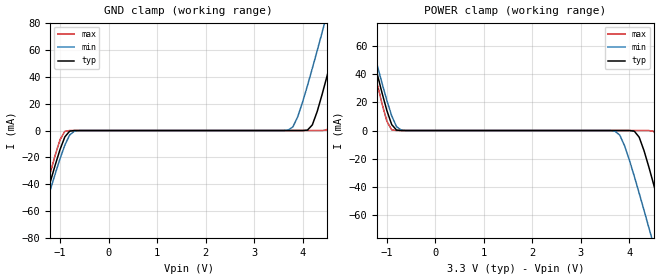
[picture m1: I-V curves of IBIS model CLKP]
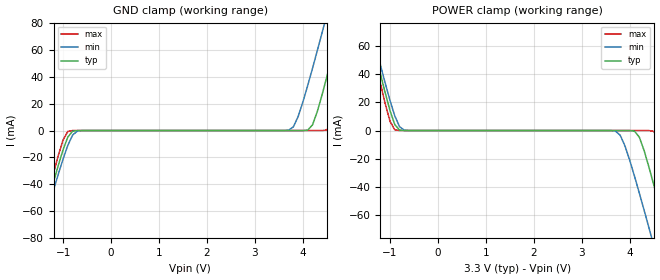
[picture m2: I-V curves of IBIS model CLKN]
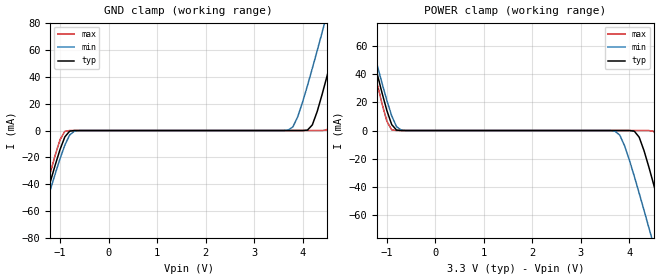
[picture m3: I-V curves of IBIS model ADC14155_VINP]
|   National Semiconductor Corporation
|   IBIS Model of ADC14155_qml
|   48 Pin LLP
[IBIS Ver]   4.0
[File name]   adc14155_qml.ibs
[File Rev]   1.0
[Date]   07/15/2009
[Source]
[Notes]   Revision History:
   Revision 1.0 : Models Generated by Shrikant GK
   Revision 1.1 : Added QML package to the IBIS file Pegah Alavi
[Disclaimer]
(C) Copyright National Semiconductor Corporation 2009
   All rights reserved
   National Semiconductor Corporation hereby grants
the user of this IBIS model a non-exclusive, nontransferable
license to use this IBIS model under the following terms.
Before using this IBIS model, the user should read this
license.  If the user does not accept these terms,  the
IBIS model should be returned to National within 30 days.
   The user is granted this license only to use the
IBIS model and is not granted rights to sell, load, rent,
lease or license the IBIS model in whole or in part, or in
modified form to anyone other than user. User may modify
the IBIS model to suit its specific applications but rights
to derivative works and such modifications shall belong to
National.
   This IBIS model is provided on an "AS IS" basis and
National makes absolutely no warranty with respect to the
information contained herein.NATIONAL DISCLAIMS AND CUSTOMER
WAIVES ALL WARRANTIES, EXPRESS OR IMPLIED, INCLUDING
WARRANTIES OF MERCHANTABILITY OR FITNESS FOR A PARTICULAR
PURPOSE. The entire risk as to quality and performance is
with the Customer. ACCORDINGLY, IN NO EVENT SHALL THE
COMPANY BE LIABLE FOR ANY DAMAGES, WHETHER IN CONTRACT OR
TORT,INCLUDING ANY LOST PROFITS OR OTHER INCIDENTAL,
CONSEQUENTIAL, EXEMPLARY, OR PUNITIVE DAMAGES ARISING OUT
OF THE USE OR APPLICATION OF THE IBIS model provided in
this package.Further, National reserves the right to make
changes without notice to any product herein to improve
reliability, function, or design. National does not convey
any license under patent rights or any other intellectual
property rights, including those of third parties.
   National is not obligated to provide maintenance or support
for the licensed IBIS model.
[Copyright]   Copyright 2009, National Semiconductor, All Rights Reserved
[Component]   ADC14155_qml
[Manufacturer]  National Semiconductor Corp
[Package]
|   typ   min   max
R_pkg   0   0   0
L_pkg   0   0   0
C_pkg   0   0   0
[Pin]   signal_name  model_name   R_pin   L_pin   C_pin
1   VA   POWER
2   AGND   GND
3   VIN-   ADC14155_VINN
4   VIN+   ADC14155_VINP
5   AGND   GND
6   VA   POWER
7   PD   NC
8   CLK_SEL   NC
9   VA   POWER
10   AGND   GND
11   CLK+   CLKP
12   CLK-   CLKN
13   VD   POWER
14   DGND   GND
15   VDR   POWER
16   DRGND   GND
17   D0   ADC14155_D0
18   D1   ADC14155_D0
19   D2   ADC14155_D0
20   D3   ADC14155_D0
21   D4   ADC14155_D0
22   D5   ADC14155_D0
23   D6   ADC14155_D0
24   D7   ADC14155_D0
25   VDR   POWER
26   DRGND   GND
27   D8   ADC14155_D0
28   D9   ADC14155_D0
29   D10   ADC14155_D0
30   D11   ADC14155_D0
31   D12   ADC14155_D0
32   D13   ADC14155_D0
33   OVR   NC
34   DRDY   ADC14155_D0
35   DRGND   GND
36   VDR   POWER
37   VA   POWER
38   AGND   GND
39   AGND   GND
40   VA   POWER
41   VA   POWER
42   AGND   GND
43   VRP   NC
44   VRN   NC
45   VRM   NC
46   VREF   NC
47   AGND   GND
48   VA   POWER
49   DAP   GND
[Diff_pin]   inv_pin   vdiff   tdelay_typ   tdelay_min   tdelay_max
| The '+' pin is Diff_pin and the '-' pin is the inv_pin
4   3   50m   0   0   0
|Electrical package information will overide all the default values.
[Package Model] ADC14155W_QML
|   Package Model
[Define Package Model]  ADC14155W_QML
[Manufacturer]   NSC
[Description]   none
[OEM]   NA
[Number Of Pins]   21
[Pin Numbers]
10   | 10 = B10
11   | 11 = B11
12   | 12 = B12
17   | 17 = B17
18   | 18 = B18
19   | 19 = B19
20   | 20 = B20
21   | 21 = B21
22   | 22 = B22
23   | 23 = B23
24   | 24 = B24
25   | 25 = B25
26   | 26 = B26
27   | 27 = B27
28   | 28 = B28
30   | 30 = B30
31   | 31 = B31
32   | 32 = B32
33   | 33 = B33
34   | 34 = B34
35   | 35 = B35
[Model Data]
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[End Model Data]
[End Package Model]
| Models and submodels in the file (5): CLKP (Input), CLKN (Input), ADC14155_VINP (Input), ADC14155_VINN (Input), ADC14155_D0 (Output)
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|   Input driver CLKP
[Model]   CLKP
Model_type Input
Polarity Non-Inverting
Vinh=2.0
Vinl=0.8
C_comp   776.6f   764.4f   787.6f
|   TYP   MIN   MAX
[Temperature Range]  25   85   -40
[Voltage Range]   3.3   3.0   3.6
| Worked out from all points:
|   GND clamp passes 1 mA (typ) near -0.81 V on its own axis
|   POWER clamp passes 1 mA (typ) near -0.82 V on its own axis
[GND Clamp]
|V(groundclamp)   I(typ)   I(min)   I(max)
-3.3V     -322.4mA   -312.6mA   -335.1mA
-1.5V     -77.49mA   -81.34mA   -73.54mA
-1.1V     -25.94mA   -32.53mA   -18.6mA
-900mV    -4.742mA   -10.9mA    -604uA
-600mV    -278.4nA   -17.67uA   -369.6pA
3.7V      84.77pA    241.1uA    8.991pA
3.9V      166.1nA    10.36mA    9.951pA
4.2V      4.188mA    46.42mA    221.4pA
4.5V      40.21mA    86.59mA    437.8uA
4.8V      82.74mA    127.8mA    33.34mA
5.1V      126.5mA    169.5mA    78.82mA
6.5V      334.4mA    366.6mA    299.9mA
[POWER Clamp]
|V(PowerClamp)   I(typ)   I(min)   I(max)
-3.3V     349.4mA    338.3mA    315.9mA
-1.5V     82.74mA    86.59mA    78.82mA
-1.4V     68.37mA    73.03mA    63.43mA
-900mV    4.188mA    10.36mA    437.8uA
-700mV    7.783uA    241.1uA    28.92nA
3.7V      -141.7pA   -368.4uA   -7.681pA
3.9V      -278.4nA   -10.9mA    -8.642pA
4.2V      -4.742mA   -44.39mA   -369.6pA
4.5V      -38.39mA   -81.34mA   -604uA
4.8V      -77.49mA   -119.2mA   -31.74mA
5.1V      -117.7mA   -157.5mA   -73.54mA
6.5V      -308.6mA   -312.6mA   -276.5mA
|   Input driver CLKN
[Model]   CLKN
Model_type Input
Polarity Inverting
Vinh=2.0
Vinl=0.8
C_comp   776.6f   764.4f   787.6f
|   TYP   MIN   MAX
[Temperature Range]   25   85   -40
[Voltage Range]   3.3   3.0   3.6
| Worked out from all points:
|   GND clamp passes 1 mA (typ) near -0.81 V on its own axis
|   POWER clamp passes 1 mA (typ) near -0.82 V on its own axis
[GND Clamp]
|V(groundclamp)   I(typ)   I(min)   I(max)
-3.3V     -322.4mA   -312.6mA   -335.1mA
-1.5V     -77.49mA   -81.34mA   -73.54mA
-1.1V     -25.94mA   -32.53mA   -18.6mA
-900mV    -4.742mA   -10.9mA    -604uA
-600mV    -278.4nA   -17.67uA   -369.6pA
3.7V      84.77pA    241.1uA    8.991pA
3.9V      166.1nA    10.36mA    9.951pA
4.2V      4.188mA    46.42mA    221.4pA
4.5V      40.21mA    86.59mA    437.8uA
4.8V      82.74mA    127.8mA    33.34mA
5.1V      126.5mA    169.5mA    78.82mA
6.5V      334.4mA    366.6mA    299.9mA
[POWER Clamp]
|V(PowerClamp)   I(typ)   I(min)   I(max)
-3.3V     349.4mA    338.3mA    315.9mA
-1.5V     82.74mA    86.59mA    78.82mA
-1.4V     68.37mA    73.03mA    63.43mA
-900mV    4.188mA    10.36mA    437.8uA
-700mV    7.783uA    241.1uA    28.92nA
3.7V      -141.7pA   -368.4uA   -7.681pA
3.9V      -278.4nA   -10.9mA    -8.642pA
4.2V      -4.742mA   -44.39mA   -369.6pA
4.5V      -38.39mA   -81.34mA   -604uA
4.8V      -77.49mA   -119.2mA   -31.74mA
5.1V      -117.7mA   -157.5mA   -73.54mA
6.5V      -308.6mA   -312.6mA   -276.5mA
|   Model of Differential Input ADC14155_VINP
[Model]   ADC14155_VINP
Model_type Input
Polarity Non-Inverting
Vinh=2.0
Vinl=1.0
C_comp   776.6f   764.4f   787.6f
|   TYP   MIN   MAX
[Temperature Range]  25   85   -40
[Voltage Range]   3.3   3.0   3.6
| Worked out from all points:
|   GND clamp passes 1 mA (typ) near -0.81 V on its own axis
|   POWER clamp passes 1 mA (typ) near -0.82 V on its own axis
[GND Clamp]
|V(groundclamp)   I(typ)   I(min)   I(max)
-3.3V     -322.4mA   -312.6mA   -335.1mA
-1.5V     -77.49mA   -81.34mA   -73.54mA
-1.1V     -25.94mA   -32.53mA   -18.6mA
-900mV    -4.742mA   -10.9mA    -604uA
-600mV    -278.4nA   -17.67uA   -369.6pA
3.7V      84.77pA    241.1uA    8.991pA
3.9V      166.1nA    10.36mA    9.951pA
4.2V      4.188mA    46.42mA    221.4pA
4.5V      40.21mA    86.59mA    437.8uA
4.8V      82.74mA    127.8mA    33.34mA
5.1V      126.5mA    169.5mA    78.82mA
6.5V      334.4mA    366.6mA    299.9mA
[POWER Clamp]
|V(PowerClamp)   I(typ)   I(min)   I(max)
-3.3V     349.4mA    338.3mA    315.9mA
-1.5V     82.74mA    86.59mA    78.82mA
-1.4V     68.37mA    73.03mA    63.43mA
-900mV    4.188mA    10.36mA    437.8uA
-700mV    7.783uA    241.1uA    28.92nA
3.7V      -141.7pA   -368.4uA   -7.681pA
3.9V      -278.4nA   -10.9mA    -8.642pA
4.2V      -4.742mA   -44.39mA   -369.6pA
4.5V      -38.39mA   -81.34mA   -604uA
4.8V      -77.49mA   -119.2mA   -31.74mA
5.1V      -117.7mA   -157.5mA   -73.54mA
6.5V      -308.6mA   -312.6mA   -276.5mA
